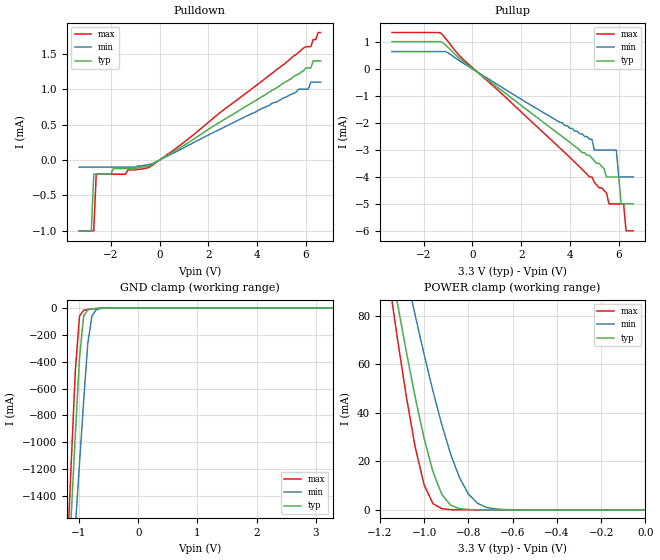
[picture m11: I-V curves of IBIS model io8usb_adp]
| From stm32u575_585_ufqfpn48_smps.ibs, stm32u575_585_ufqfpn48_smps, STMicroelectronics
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|   Model io8usb_adp
[Model]  io8usb_adp
Model_type I/O
Polarity   Non-Inverting
Enable   Active-High
Vinl =   0.990000V
Vinh =   2.310000V
Vmeas =  1.650000V
Cref =   50.000000pF
Rref =   100.000000M
Vref =   0.0V
C_comp   3.171500pF   3.148500pF   3.202800pF
[Temperature Range]   25.000000   0.140000k   -40.000000
[Pullup Reference]   3.300000V   2.700000V   3.600000V
[Pulldown Reference]   0.0V   0.0V   0.0V
[POWER Clamp Reference]   3.300000V   2.700000V   3.600000V
[GND Clamp Reference]   0.0V   0.0V   0.0V
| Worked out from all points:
|   slope of the pulldown table from 0 to 0.495 V, typ, clamps not added: 4.89 kohm
|   slope of the pullup table from 0 to 0.495 V, typ, clamps not added: 1.48 kohm
|   GND clamp passes 1 mA (typ) near -0.53 V on its own axis
|   POWER clamp passes 1 mA (typ) near -0.85 V on its own axis
[Pulldown]
|Voltage   I(typ)   I(min)   I(max)
-3.3V     -1mA       -100uA     -1mA
-2.8V     -1mA       -100uA     -1mA
-2.7V     -200uA     -100uA     -1mA
-2.6V     -200uA     -100uA     -200uA
-1.4V     -120uA     -100uA     -200uA
-1.3V     -120uA     -100uA     -140uA
-400mV    -78.2uA    -60.57uA   -96.71uA
5.7V      1.21mA     1mA        1.52mA
6.1V      1.3mA      1mA        1.6mA
6.2V      1.3mA      1.1mA      1.6mA
6.3V      1.4mA      1.1mA      1.7mA
6.6V      1.4mA      1.1mA      1.8mA
[Pullup]
|Voltage   I(typ)   I(min)   I(max)
-3.3V     1.02mA     650uA      1.36mA
-1.3V     1.02mA     650uA      1.34mA
4.9V      -3.3mA     -2.6mA     -4mA
5V        -3.4mA     -3mA       -4.2mA
5.5V      -4mA       -3mA       -4.6mA
5.6V      -4mA       -3mA       -5mA
5.9V      -4mA       -3mA       -5mA
6V        -4mA       -4mA       -5mA
6.1V      -5mA       -4mA       -5mA
6.2V      -5mA       -4mA       -5mA
6.3V      -5mA       -4mA       -6mA
6.6V      -5mA       -4mA       -6mA
[GND_clamp]
|Voltage   I(typ)   I(min)   I(max)
-3.3V     -9.415A    -9.508A    -9.703A
-1.2V     -2.138A    -2.581A    -1.86A
-1.13V    -1.538A    -2.104A    -1.153A
-1.06V    -942.5mA   -1.629A    -463.6mA
-990mV    -370.9mA   -1.155A    -61.04mA
-920mV    -60.47mA   -689.2mA   -18.45mA
-850mV    -14.7mA    -261.7mA   -12.53mA
-780mV    -7.72mA    -59.92mA   -8.757mA
-710mV    -4.894mA   -15.16mA   -5.593mA
-640mV    -2.894mA   -5.172mA   -3.09mA
-360mV    -21.77uA   -117.9uA   -5.95uA
3.28V     0A         10.04nA    -7.986nA
[POWER_clamp]
|Voltage   I(typ)   I(min)   I(max)
-3.28V    1.355A     1.167A     1.664A
-1.16V    105.7mA    131.6mA    95.69mA
-1.12V    84.97mA    114mA      70.27mA
-1.08V    65.05mA    96.83mA    46.54mA
-1.04V    46.34mA    80.15mA    25.76mA
-1V       29.51mA    64.13mA    10.3mA
-960mV    15.69mA    48.99mA    2.571mA
-920mV    6.373mA    35.1mA     455.6uA
-840mV    490.7uA    13.24mA    11.36uA
-760mV    27.33uA    2.767mA    731.6nA
-640mV    346.7nA    134.1uA    731.6nA
0V        0A         15.13nA    0A
[Ramp]
| variable   typ   min   max
dV/dt_r  64.91993m/0.87368n  43.76131m/1.12757n  84.50971m/1.24006n
dV/dt_f  20.16000m/0.93366n  13.80000m/1.33860n  26.70000m/0.64493n
R_load = 50.000000
|End [Model] io8usb_adp
